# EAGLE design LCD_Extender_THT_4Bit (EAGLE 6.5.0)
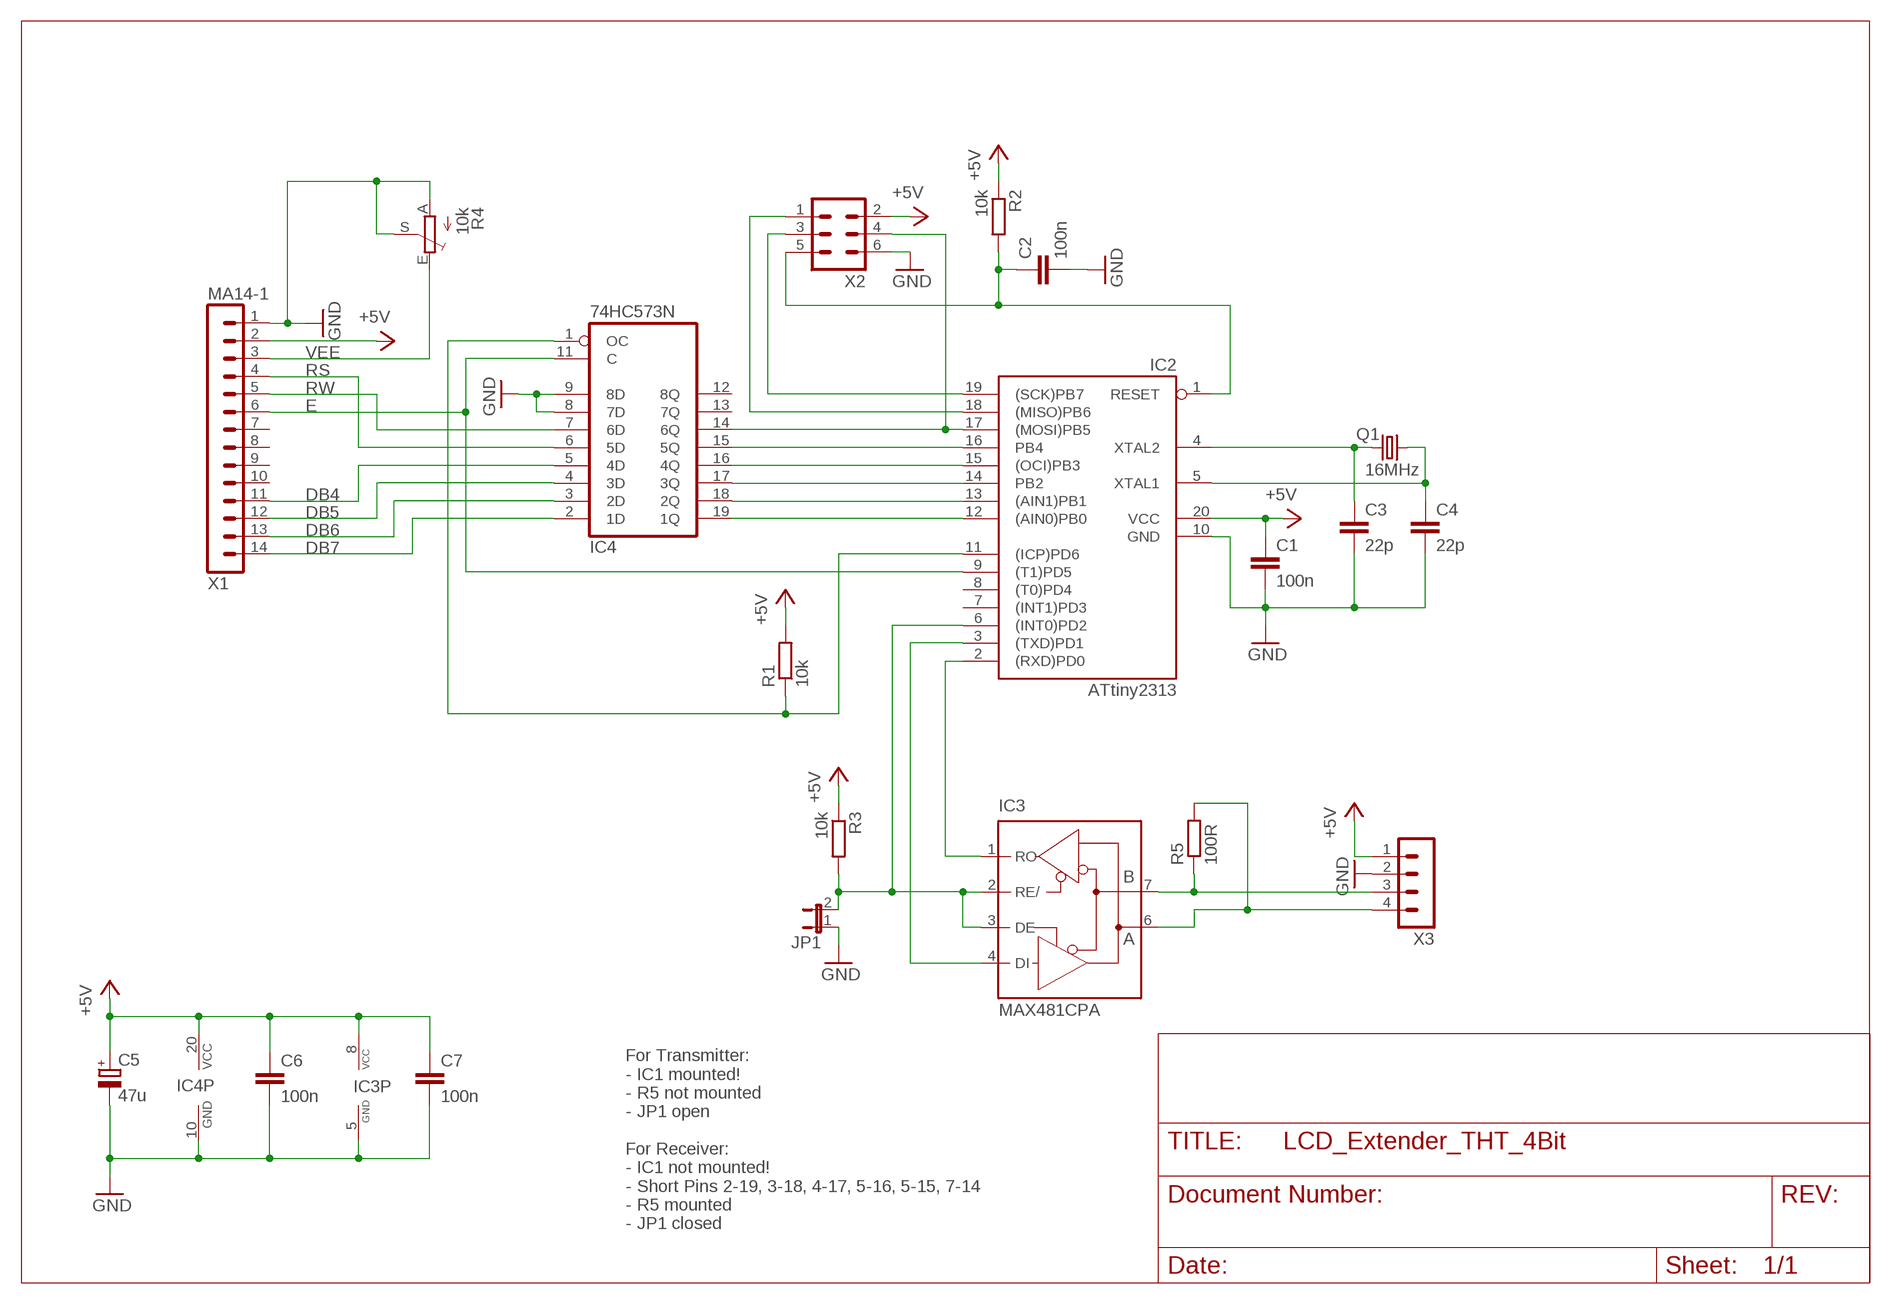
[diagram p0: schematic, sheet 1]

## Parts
C1  100n  C-EU050-024X044  [C050-024X044]
C2  100n  C-EU050-024X044  [C050-024X044]
C3  22p  C-EU050-024X044  [C050-024X044]
C4  22p  C-EU050-024X044  [C050-024X044]
C5  47u  CPOL-EUE2.5-6  [E2,5-6]
C6  100n  C-EU050-024X044  [C050-024X044]
C7  100n  C-EU050-024X044  [C050-024X044]
IC2  ATtiny2313  AT90S2313P  [DIL20]
IC3  MAX481CPA  [DIL08]
IC4  74HC573N  [DIL20]
JP1  JP1E  [JP1]
Q1  16MHz  CRYSTALHC49U-V  [HC49U-V]
R1  10k  R-EU_0207/10  [0207/10]
R2  10k  R-EU_0207/10  [0207/10]
R3  10k  R-EU_0207/10  [0207/10]
R4  10k  TRIM_EU-B25V  [B25V]
R5  100R  R-EU_0207/10  [0207/10]
X1  MA14-1  [MA14-1]
X2  ML6  [ML6]
X3  MA04-1  [MA04-1]

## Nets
+5V: C1.1 C5.+ C6.1 C7.1 IC2.20(VCC) IC3.8(VCC) IC4.20(VCC) R1.2 R2.1 R3.1 X1.2 X2.2 X3.1
DB4: IC4.5(4D) X1.11
DB5: IC4.4(3D) X1.12
DB6: IC4.3(2D) X1.13
DB7: IC4.2(1D) X1.14
E: IC2.9((T1)PD5) IC4.11(C) X1.6
GND: C1.2 C2.2 C3.2 C4.2 C5.- C6.2 C7.2 IC2.10(GND) IC3.5(GND) IC4.8(7D) IC4.9(8D) IC4.10(GND) JP1.1 R4.A R4.S X1.1 X2.6 X3.2
N$1: IC2.19((SCK)PB7) X2.3
N$2: C3.1 IC2.4(XTAL2) Q1.1
N$3: IC2.17((MOSI)PB5) IC4.14(6Q) X2.4
N$4: IC2.16(PB4) IC4.15(5Q)
N$5: IC2.15((OCI)PB3) IC4.16(4Q)
N$6: IC2.13((AIN1)PB1) IC4.18(2Q)
N$7: IC2.3((TXD)PD1) IC3.4(DI)
N$8: IC2.14(PB2) IC4.17(3Q)
N$9: C4.1 IC2.5(XTAL1) Q1.2
N$10: IC3.7(B) R5.1 X3.3
N$11: IC3.6(A) R5.2 X3.4
N$12: IC2.12((AIN0)PB0) IC4.19(1Q)
N$14: C2.1 IC2.1(RESET) R2.2 X2.5
N$15: IC2.11((ICP)PD6) IC4.1(OC) R1.1
N$16: IC2.18((MISO)PB6) X2.1
N$29: IC2.2((RXD)PD0) IC3.1(RO)
N$30: IC2.6((INT0)PD2) IC3.2(RE/) IC3.3(DE) JP1.2 R3.2
RS: IC4.6(5D) X1.4
RW: IC4.7(6D) X1.5
VEE: R4.E X1.3
Unconnected: IC2.7((INT1)PD3) IC2.8((T0)PD4) IC4.12(8Q) IC4.13(7Q) X1.7 X1.8 X1.9 X1.10

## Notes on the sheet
- For Transmitter:
  - IC1 mounted!
  - R5 not mounted
  - JP1 open
  
  For Receiver:
  - IC1 not mounted!
  - Short Pins 2-19, 3-18, 4-17, 5-16, 5-15, 7-14
  - R5 mounted
  - JP1 closed

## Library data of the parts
C1-C4 C6 C7 = rcl:C-EU: CAPACITOR, European symbol
C5 = rcl:CPOL-EU: POLARIZED CAPACITOR, European symbol
IC2 = atmel:AT90S2313: MICROCONTROLLER 2 Kbytes FLASH 128 bytes SRAM 128 bytes EEPROM UART; OC_FARNELL: unknown; OC_NEWARK: unknown
IC3 = maxim:MAX481CPA: RS485 TRANSEIVER; MPN: MAX481CPA+; OC_FARNELL: unknown; OC_NEWARK: 99K3445
IC4 = 74xx-eu:74*573: 8-bit D latch BUS DRIVER
JP1 = jumper:JP1E: JUMPER
Q1 = crystal:CRYSTAL: CRYSTAL; OC_FARNELL: 1666969; OC_NEWARK: unknown
R1-R3 R5 = rcl:R-EU_: RESISTOR, European symbol
R4 = pot:TRIM_EU-: POTENTIOMETER
X1 = Brunner:MA14-1
X2 = con-harting-ml:ML6: HARTING; OC_FARNELL: unknown; OC_NEWARK: unknown
X3 = con-lstb:MA04-1: PIN HEADER; OC_FARNELL: unknown; OC_NEWARK: unknown

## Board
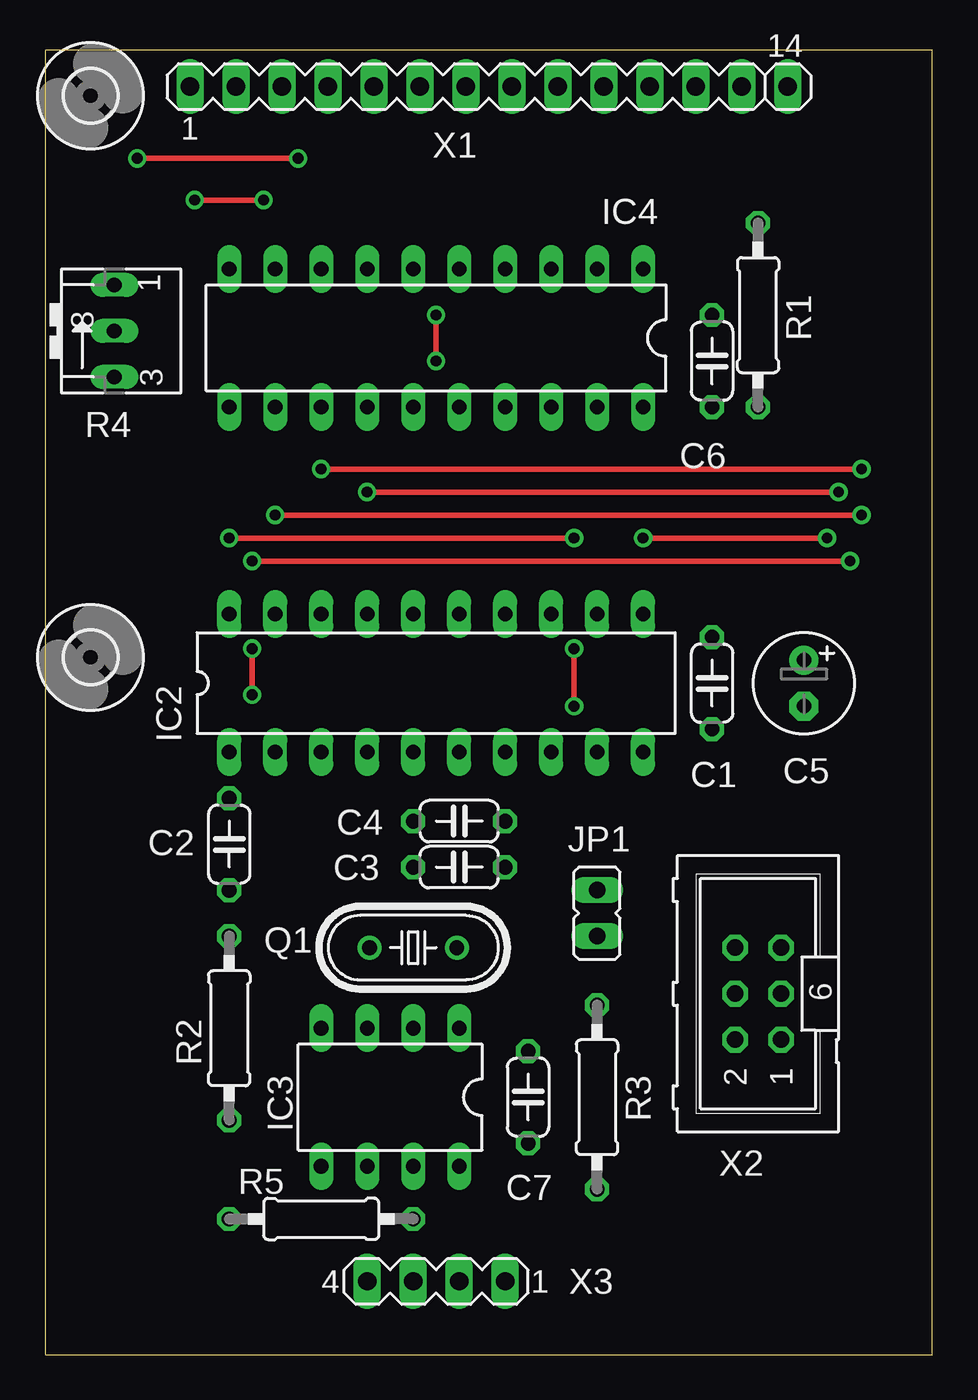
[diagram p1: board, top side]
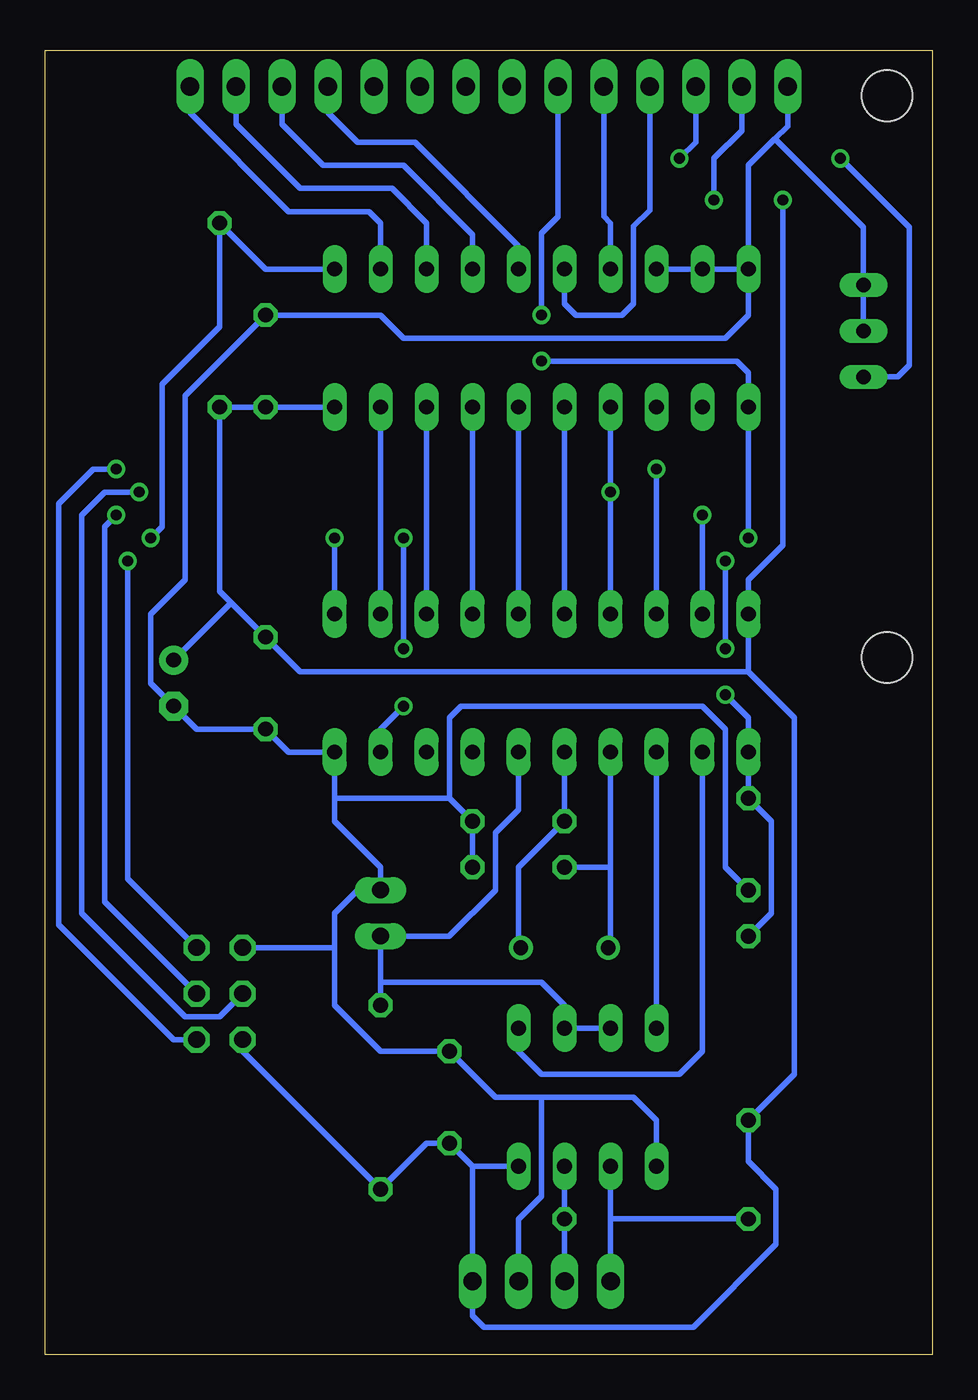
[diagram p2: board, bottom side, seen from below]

Size 49 x 72 mm. Coordinates in mm from the lower left corner, seen from the top.
Outline: 0,72 0,0 49,0 49,72 0,72
Copper layers (1*16): Top 0.035mm / dielectric 1.5mm / Bottom 0.035mm
Design rules "default *": minimum track width 10mil, minimum drill 0.6mm, track to track 0.3mm, track to pad 0.3mm, pad to pad 0.3mm, via to via 0.3mm, smd to smd 8mil, copper to edge 0.4mm, drill to drill 8mil, minimum pad ring 10mil, minimum via ring 8mil, stop-mask expansion 4mil, vias tented up to drill 0mil, thermal gap 10mil

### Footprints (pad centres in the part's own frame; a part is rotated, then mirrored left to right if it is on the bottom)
C050-024X044 = drill 0.813 octagon: 1 -2.54,0; 2 2.54,0
E2,5-6 = drill 0.813 pad 1.6: + -1.27,0 | drill 0.813 pad 1.6 octagon: - 1.27,0
DIL20 = drill 0.813 long: 1 -11.43,-3.81; 2 -8.89,-3.81; 3 -6.35,-3.81; 4 -3.81,-3.81; 5 -1.27,-3.81; 6 1.27,-3.81; 7 3.81,-3.81; 8 6.35,-3.81; 9 8.89,-3.81; 10 11.43,-3.81; 11 11.43,3.81; 12 8.89,3.81; 13 6.35,3.81; 14 3.81,3.81; 15 1.27,3.81; 16 -1.27,3.81; 17 -3.81,3.81; 18 -6.35,3.81; 19 -8.89,3.81; 20 -11.43,3.81
DIL08 = drill 0.813 long: 1 -3.81,-3.81; 2 -1.27,-3.81; 3 1.27,-3.81; 4 3.81,-3.81; 5 3.81,3.81; 6 1.27,3.81; 7 -1.27,3.81; 8 -3.81,3.81
JP1 = drill 0.914 long: 1 0,-1.27; 2 0,1.27
HC49U-V = drill 0.813: 1 -2.413,0; 2 2.413,0
0207/10 = drill 0.813 octagon: 1 -5.08,0; 2 5.08,0
B25V = drill 0.813 long: A 2.54,0.635; E -2.54,0.635; S 0,0.635
2,8 = hole 2.8: 0,0
MA14-1 = drill 1.016 long: 1 -16.51,0; 2 -13.97,0; 3 -11.43,0; 4 -8.89,0; 5 -6.35,0; 6 -3.81,0; 7 -1.27,0; 8 1.27,0; 9 3.81,0; 10 6.35,0; 11 8.89,0; 12 11.43,0; 13 13.97,0; 14 16.51,0
ML6 = drill 0.914 octagon: 1 -2.54,-1.27; 2 -2.54,1.27; 3 0,-1.27; 4 0,1.27; 5 2.54,-1.27; 6 2.54,1.27
MA04-1 = drill 1.016 long: 1 -3.81,0; 2 -1.27,0; 3 1.27,0; 4 3.81,0

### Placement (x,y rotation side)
C1  36.83,37.08 270 top
C2  10.16,28.18 270 top
C3  22.86,26.91 0 top
C4  22.86,29.45 0 top
C5  41.91,37.08 270 top
C6  36.83,54.85 90 top
C7  26.67,14.21 90 top
IC2  21.59,37.08 0 top
IC3  19.05,14.21 180 top
IC4  21.59,56.12 180 top
JP1  30.48,24.38 180 top
Q1  20.32,22.47 0 top
R1  39.37,57.4 270 top
R2  10.16,18.02 90 top
R3  30.48,14.21 90 top
R4  4.45,56.52 90 top
R5  15.24,7.49 180 top
U$1  [2,8]  2.5,69.5 0 top
U$2  [2,8]  2.5,38.5 0 top
X1  24.5,70 0 top
X2  39.37,19.93 90 top
X3  21.59,4.05 180 top

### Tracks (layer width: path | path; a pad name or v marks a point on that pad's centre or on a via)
+5V  (via drill 0.6)
  Top 0.305: v12.06,63.74 v8.26,63.74
  Bottom 0.305: 10.16,37.71 34.92,37.71 C1.1 38.73,41.52 | 10.16,37.71 IC2.20 10.16,42.79 8.26,44.7 v8.26,63.74 | IC3.8 25.4,10.4 | 25.4,10.4 C7.1 27.94,11.68 R3.1 38.1,16.75 X2.2 | 25.4,10.4 X3.1 25.4,2.15 24.77,1.51 13.72,1.51 13.71,1.52 13.21,1.52 8.64,6.1 8.64,9.14 10.16,10.67 R2.1 7.62,15.48 7.62,35.17 10.16,37.71 | IC4.20 C6.1 R1.2 39.37,42.16 38.73,41.52 | C5.+ 38.73,41.52 | X1.2 10.53,67.58 12.06,66.04 v12.06,63.74
DB4
  Bottom 0.305: IC4.5 22.86,61.2 28.57,66.92 31.75,66.92 33.39,68.56 X1.11
DB5
  Bottom 0.305: IC4.4 25.4,61.84 29.21,65.65 33.66,65.65 35.93,67.92 X1.12
DB6
  Bottom 0.305: IC4.3 27.94,62.48 29.84,64.38 34.92,64.38 38.47,67.92 X1.13
DB7
  Bottom 0.305: IC4.2 30.48,62.48 31.11,63.11 35.56,63.11 41.01,68.56 X1.14
E  (via drill 0.6)
  Top 0.305: v29.21,45.09 v10.16,45.09 | v21.59,54.85 v21.59,57.4 | v29.21,35.8 v29.21,38.98
  Bottom 0.305: v10.16,45.09 IC4.11 10.16,54.22 10.79,54.85 v21.59,54.85 | v21.59,57.4 21.59,61.92 20.69,62.82 X1.6 | IC2.9 30.48,34.53 v29.21,35.8 | v29.21,38.98 v29.21,45.09
GND
  Bottom 0.305: C3.2 C4.2 26.67,30.73 | 33.02,30.73 33.02,29.45 30.48,26.91 JP1.1 31.75,25.64 33.02,24.38 33.02,22.47 | 33.02,30.73 IC2.10 35.56,33.27 C1.2 40.64,34.53 C5.- 43.18,37.08 43.18,40.88 41.27,42.79 41.27,52.95 C6.2 30.48,57.4 29.21,56.12 11.43,56.12 10.16,57.4 IC4.10 | 21.59,14.21 24.13,14.21 C7.2 30.48,16.75 33.02,19.3 33.02,22.47 | 21.59,14.21 16.51,14.21 15.24,12.95 IC3.5 | X3.2 22.86,7.48 21.59,8.75 21.59,14.21 | 26.67,30.73 26.67,35.17 26.04,35.8 12.7,35.8 11.43,34.53 11.43,26.91 C2.2 | X2.6 33.02,22.47 | IC4.10 10.16,65.65 8.7,67.11 | IC4.8 IC4.9 IC4.10 | 33.02,30.73 26.67,30.73 | X1.1 7.99,67.82 8.7,67.11 | R4.S R4.A 3.81,62.23 8.7,67.11
N$1  (via drill 0.6)
  Top 0.305: v45.09,46.35 v12.7,46.35
  Bottom 0.305: IC2.19 v12.7,46.35 | X2.3 45.72,25.01 45.72,45.72 v45.09,46.35
N$2
  Bottom 0.305: IC2.4 17.78,26.91 | 17.78,26.91 17.78,22.6 Q1.1 | C3.1 17.78,26.91
N$3  (via drill 0.6)
  Top 0.305: v43.81,47.62 v17.78,47.62
  Bottom 0.305: IC2.17 v17.78,47.62 IC4.14 | X2.4 39.37,18.66 41.27,18.66 46.99,24.38 46.99,46.35 45.72,47.62 v43.81,47.62
N$4
  Bottom 0.305: IC4.15 IC2.16
N$5
  Bottom 0.305: IC2.15 IC4.16
N$6
  Bottom 0.305: IC2.13 IC4.18
N$7
  Bottom 0.305: IC2.3 IC3.4
N$8
  Bottom 0.305: IC4.17 IC2.14
N$9
  Bottom 0.305: IC2.5 C4.1 22.86,26.91 22.86,22.6 Q1.2
N$10
  Bottom 0.305: X3.3 R5.1 IC3.7
N$11
  Bottom 0.305: X3.4 17.78,7.62 | 17.78,7.62 IC3.6 | R5.2 17.65,7.49 17.78,7.62
N$12
  Bottom 0.305: IC4.19 IC2.12
N$14  (via drill 0.6)
  Top 0.305: v44.45,43.81 v11.43,43.81 | v11.43,38.98 v11.43,36.44
  Bottom 0.305: R2.2 8.89,24.38 8.89,29.45 C2.1 IC2.1 10.16,35.17 v11.43,36.44 | v44.45,43.81 44.45,26.28 X2.5 | v11.43,43.81 v11.43,38.98
N$15  (via drill 0.6)
  Top 0.305: v33.02,45.09 v43.18,45.09
  Bottom 0.305: IC4.1 36.83,59.94 R1.1 39.37,56.76 42.55,53.59 42.55,45.72 v43.18,45.09 | IC2.11 v33.02,45.09
N$16  (via drill 0.6)
  Top 0.305: v45.09,48.9 v15.24,48.9
  Bottom 0.305: v15.24,48.9 IC2.18 | X2.1 41.91,17.39 48.26,23.74 48.26,46.99 46.35,48.9 v45.09,48.9
N$29
  Bottom 0.305: IC2.2 12.7,16.75 13.97,15.48 21.59,15.48 22.86,16.75 IC3.1
N$30
  Bottom 0.305: IC3.3 IC3.2 20.32,19.3 21.59,20.57 30.47,20.57 30.48,20.57 | 30.48,20.57 JP1.2 26.71,23.11 25.44,24.38 25.4,24.38 24.13,25.64 24.13,28.82 22.86,30.09 IC2.6 | 30.48,20.57 R3.2
RS
  Bottom 0.305: IC4.6 20.32,58.03 19.68,57.4 17.14,57.4 16.51,58.03 16.51,62.28 15.61,63.19 X1.4
RW
  Bottom 0.305: IC4.7 17.78,62.48 18.15,62.84 X1.5
VEE  (via drill 0.6)
  Top 0.305: v13.97,66.04 v5.08,66.04
  Bottom 0.305: X1.3 13.07,66.94 v13.97,66.04 | v5.08,66.04 1.27,62.23 1.27,54.61 1.91,53.98 R4.E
